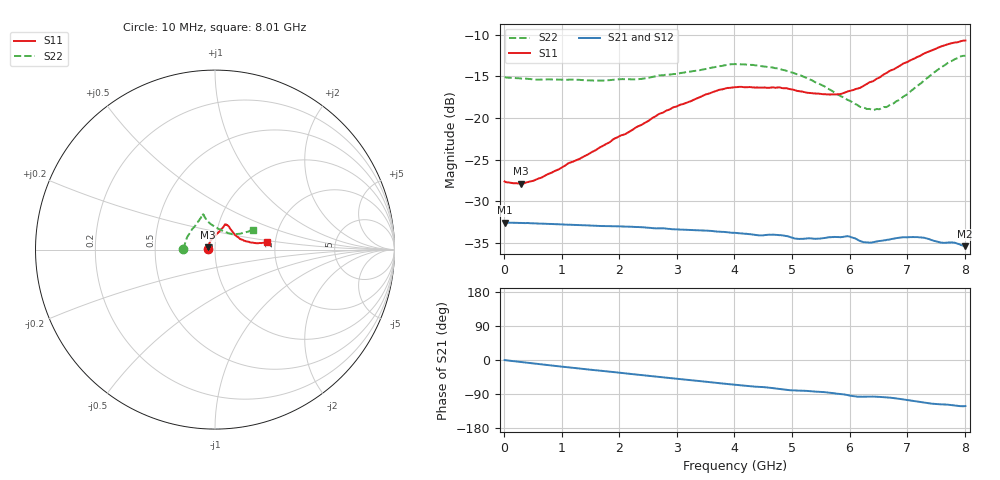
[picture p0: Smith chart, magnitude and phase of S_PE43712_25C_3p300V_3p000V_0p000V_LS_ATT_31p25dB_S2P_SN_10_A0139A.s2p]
! DEVICE ID: PE43712
! File Path: z:\PE43713\PE43713_CHAR_NOM_04292014\AMB\3p300\LS_ATT_31p25dB\PE43713_AMB_3p300V_3p000V_0p000V_LS_ATT_31p25dB_S2P_SN_10_A0139A.s2p
! Serial: 10
! Lot: A0139A
! Temp: 25C
! VDD: 3.300
! VSS: 0.000
! Control_Hi: 3.000
! Control_Lo: 0.000
! Attenuation Step: 31.25dB
! Port 1: RF1
! Port 2: RF2
! ThroughPath:1-2
! IDD: 0.0001459008
! ISS: -9.71e-008
#  Hz  S  RI  R  50
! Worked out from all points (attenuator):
!   801 points, 10 MHz to 8.01 GHz, reference 50 ohm
!   highest |S21| = -32.52 dB at 10 MHz (marker M1); lowest = -35.4 dB at 8 GHz (marker M2)
!   lowest |S11| = -27.9 dB at 290 MHz (marker M3), VSWR 1.08, Z = 46.3 + j1.23 ohm
!   |S11| at or under -10 dB: start of sweep to end of sweep
!   |S22| runs from -19.0 to -12.5 dB; largest |S21 - S12| = 9.9e-05
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1e7  -0.0417 0.0009  0.0237 -0.000116  0.0236 -9.91e-05  -0.1759 0.00122
2.9e8  -0.0381 0.0133  0.0234 -0.00217  0.0234 -0.00217  -0.1717 0.0184
6.5e8  -0.0338 0.0281  0.0228 -0.00468  0.0228 -0.00467  -0.1653 0.0391
1.35e9  -0.021 0.0541  0.021 -0.00897  0.021 -0.00899  -0.1508 0.0761
2.3e9  0.01 0.0877  0.0174 -0.0138  0.0174 -0.0138  -0.1164 0.1248
2.68e9  0.025 0.1024  0.0156 -0.0153  0.0156 -0.0153  -0.1002 0.1493
3.5e9  0.0484 0.1298  0.0114 -0.0178  0.0114 -0.0178  -0.0769 0.1811
4.01e9  0.0582 0.1416  0.00857 -0.0186  0.00855 -0.0186  -0.0739 0.1973
4.76e9  0.0721 0.1345  0.0048 -0.0193  0.00482 -0.0193  -0.0604 0.1888
5.09e9  0.0821 0.1201  0.00311 -0.0186  0.00314 -0.0187  -0.0529 0.1755
5.35e9  0.0911 0.1073  0.00234 -0.0188  0.00234 -0.0188  -0.0459 0.1619
5.78e9  0.112 0.0819  0.000392 -0.0194  0.000408 -0.0194  -0.0178 0.1385
5.97e9  0.1257 0.0714  -0.00094 -0.0195  -0.000919 -0.0195  -0.00198 0.1283
6.2e9  0.1414 0.0584  -0.00224 -0.0181  -0.00217 -0.0181  0.0215 0.1143
6.41e9  0.1584 0.0514  -0.00204 -0.0179  -0.00201 -0.0179  0.0446 0.1023
6.68e9  0.1852 0.0435  -0.003 -0.0184  -0.00296 -0.0184  0.0763 0.091
6.87e9  0.2017 0.039  -0.00421 -0.0187  -0.00422 -0.0187  0.0951 0.087
7.2e9  0.2315 0.0358  -0.00664 -0.0181  -0.00662 -0.0181  0.1312 0.0879
7.69e9  0.2733 0.039  -0.00836 -0.0158  -0.0083 -0.0158  0.1869 0.101
7.82e9  0.2805 0.0408  -0.009 -0.0155  -0.00896 -0.0155  0.1982 0.1064
8e9  0.2882 0.0427  -0.00899 -0.0145  -0.00893 -0.0145  0.2094 0.1095
8.01e9  0.2887 0.0433  -0.00893 -0.0146  -0.00886 -0.0146  0.2101 0.1096
